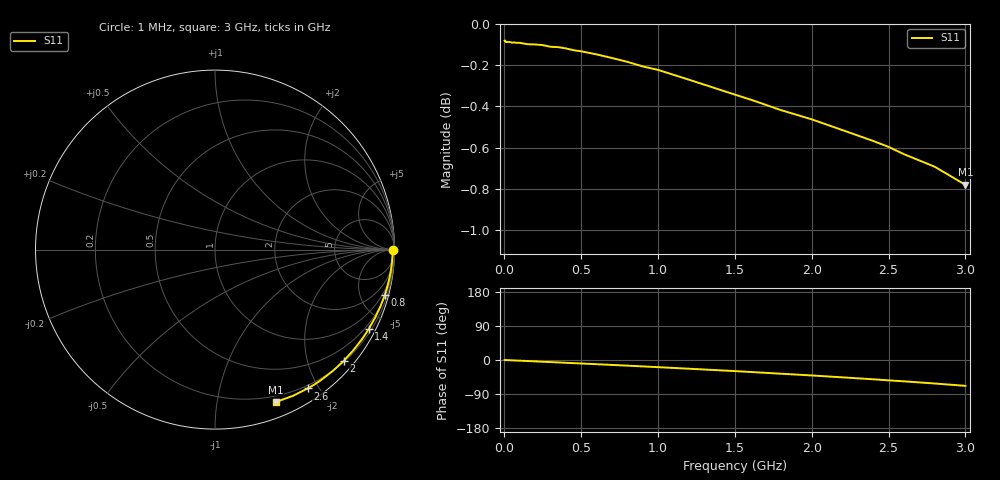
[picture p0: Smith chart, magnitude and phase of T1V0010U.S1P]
! SIEMENS Small Signal Semiconductors
! BAT68-04
! Si Schottky Diode (2 diodes in series, pin 3 open) in SOT23
! IF = 0.01 mA
! S-Parameters:  August  1994
# GHz  S  MA  R  50
!  f  S11
! GHz  MAG  ANG
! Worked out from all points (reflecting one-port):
!   33 points, 1 MHz to 3 GHz, reference 50 ohm
!   lowest |S11| = -0.8 dB at 3 GHz (marker M1), VSWR 22.26, Z = 7.12 - j73.4 ohm
!   phase of S11 starts at 0 deg and turns -68 deg over the sweep
!   S11 on the Smith chart (normalised r, x): 1 MHz: open; 800 MHz: 0.62, -7.60; 1.4 GHz: 0.33, -4.11; 2 GHz: 0.22, -2.67; 2.6 GHz: 0.16, -1.86; 3 GHz: 0.14, -1.47
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0.001  0.9908 0.0
0.003  0.9909 0.0
0.01  0.99 -0.2
0.03  0.9901 -0.5
0.08  0.9896 -1.5
0.1  0.9896 -1.8
0.15  0.9888 -2.7
0.2  0.9887 -3.7
0.25  0.9883 -4.6
0.35  0.9872 -6.4
0.4  0.9865 -7.4
0.5  0.9849 -9.2
0.6  0.9832 -11.1
0.7  0.9812 -13.0
0.8  0.9791 -14.9
1  0.9747 -18.9
1.2  0.9694 -23.0
1.4  0.964 -27.2
1.5  0.9613 -29.3
1.6  0.9587 -31.6
1.8  0.953 -36.2
2  0.9481 -40.8
2.2  0.9424 -45.8
2.4  0.9367 -50.9
2.5  0.9336 -53.7
2.6  0.9298 -56.3
2.8  0.9233 -62.0
3  0.914 -68.2
